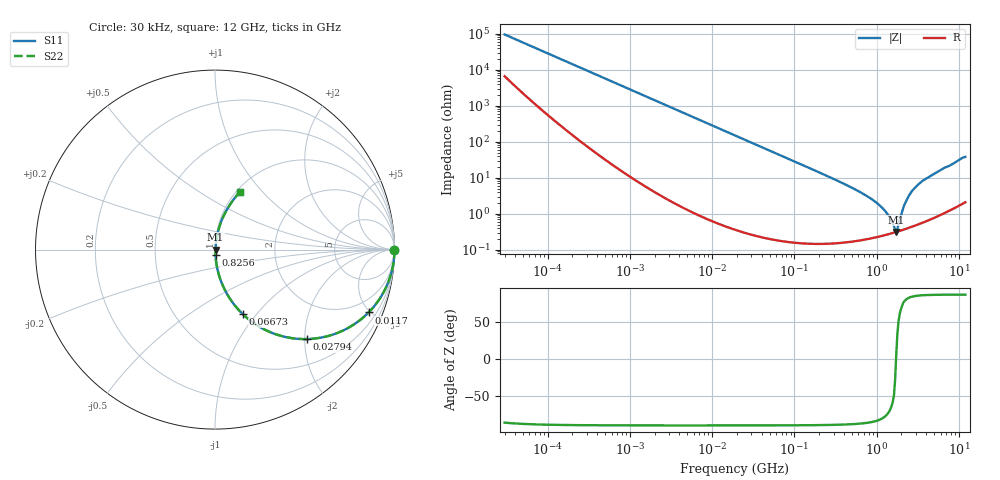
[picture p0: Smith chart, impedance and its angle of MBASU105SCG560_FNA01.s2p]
! MBASU105SCG560_FNA01  S-PARAMETER MODEL  ( General Type )
! Model Generated by TAIYO YUDEN Corporation (http://www.ty-top.com)
! Version 1.0
! TAIYO YUDEN Control No. 130207
! Copyright(c) 2013 TAIYO YUDEN CO.,LTD. All Rights Reserved.
! Product Description (link to TY-COMPAS)
! https://ds.yuden.co.jp/TYCOMPAS/or/detail?pn=MBASU105SCG560JFNA01&u=M
! Products Name : Multilayer Ceramic Capacitors
! Characteristics :
!  Capacitance : 56 pF , Rated Voltage : 50V , TCC : CG / C0G
!  Case Size : 1.0 x 0.5 / 0.039 x 0.02 [mm/inch] , Thickness : 0.5 / 0.02 [mm/inch]
!  (Conditions: Temperature = 25 degC , DC Bias Current/Voltage = 0A / 0V)
! External Node Assignments :
!  1  o---| |---o  2
! GND o---------o GND
! Frequency Range : 30000Hz  -  12GHz  [ 401 STEP ]
# MHz S RI R 50
! Freq[MHz].  S11 Real  S11 Imag  S21 Real  S21 Imag  S12 Real  S12 Imag  S22 Real  S22 Imag
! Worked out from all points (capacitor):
!   401 points, 30 kHz to 12 GHz, reference 50 ohm
!   read as one part in series: C = 55.7 pF near 32 kHz
!   lowest |Z| = 315 mohm at 1.733 GHz (marker M1)
!   series resonance near 1.724 GHz, so ESL is about 150 pH
!   S11 on the Smith chart (normalised r, x): 30 kHz: open; 11.7 MHz: 1.01, -4.89; 27.94 MHz: 1.01, -2.05; 66.73 MHz: 1.00, -0.86; 825.6 MHz: 1.00, -0.06; 12 GHz: 1.04, +0.76
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0.03  0.9999 -0.00104  7.35e-05 0.00104  7.35e-05 0.00104  0.9999 -0.00104
0.260295  0.9998 -0.0091  0.000162 0.0091  0.000162 0.0091  0.9998 -0.0091
2.258455  0.9936 -0.0785  0.00641 0.0785  0.00641 0.0785  0.9936 -0.0785
6.13721  0.9555 -0.205  0.0445 0.205  0.0445 0.205  0.9555 -0.205
11.69699  0.8561 -0.3499  0.1439 0.3499  0.1439 0.3499  0.8561 -0.3499
18.97367  0.6938 -0.4597  0.3062 0.4597  0.3062 0.4597  0.6938 -0.4597
27.93914  0.5114 -0.4985  0.4886 0.4985  0.4886 0.4985  0.5114 -0.4985
66.73476  0.1558 -0.3606  0.8442 0.3606  0.8442 0.3606  0.1558 -0.3606
164.6252  0.0302 -0.1668  0.9698 0.1668  0.9698 0.1668  0.0302 -0.1668
447.3588  0.0052 -0.0597  0.9948 0.0597  0.9948 0.0597  0.0052 -0.0597
825.5698  0.00279 -0.0274  0.9972 0.0274  0.9972 0.0274  0.00279 -0.0274
1139.739  0.00263 -0.0152  0.9974 0.0152  0.9974 0.0152  0.00263 -0.0152
1428.372  0.0028 -0.00773  0.9972 0.00773  0.9972 0.00773  0.0028 -0.00773
1625.032  0.003 -0.00344  0.997 0.00344  0.997 0.00344  0.003 -0.00344
1733.294  0.00312 0.000345  0.9969 -0.000345  0.9969 -0.000345  0.00312 0.000345
1848.769  0.00328 0.00405  0.9967 -0.00405  0.9967 -0.00405  0.00328 0.00405
2103.309  0.00378 0.014  0.9962 -0.014  0.9962 -0.014  0.00378 0.014
2316.96  0.00443 0.0239  0.9956 -0.0239  0.9956 -0.0239  0.00443 0.0239
2998.885  0.0078 0.055  0.9922 -0.055  0.9922 -0.055  0.0078 0.055
3758.338  0.013 0.0844  0.987 -0.0844  0.987 -0.0844  0.013 0.0844
6096.395  0.036 0.1603  0.964 -0.1603  0.964 -0.1603  0.036 0.1603
12000  0.1397 0.3203  0.8603 -0.3203  0.8603 -0.3203  0.1397 0.3203
